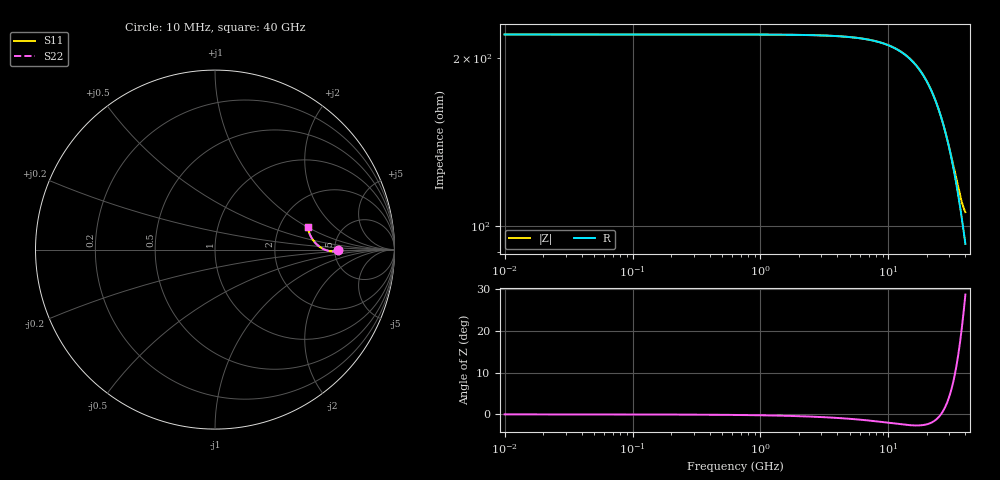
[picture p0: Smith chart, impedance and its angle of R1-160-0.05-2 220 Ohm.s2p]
!version-1
!date-03.2021
# MHz S RI R 50
!Freq ReS11 ImS11 ReS21 ImS21 ReS12 ImS12 ReS22 ImS22
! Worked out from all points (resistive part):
!   801 points, 10 MHz to 40 GHz, reference 50 ohm
!   read as one part in series: R = 220 ohm at 210 MHz
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10  0.6875 -8.09e-06  0.3125 8.07e-06  0.3125 8.07e-06  0.6875 -8.16e-06
3410  0.6864 -0.00274  0.3136 0.00274  0.3136 0.00274  0.6864 -0.00277
6710  0.6834 -0.00532  0.3166 0.0053  0.3166 0.0053  0.6834 -0.00537
10060  0.6779 -0.0077  0.3221 0.00768  0.3221 0.00768  0.6779 -0.00777
13360  0.67 -0.00954  0.33 0.00951  0.33 0.00951  0.67 -0.00963
15060  0.6648 -0.0101  0.3352 0.0101  0.3352 0.0101  0.6648 -0.0103
16710  0.659 -0.0104  0.341 0.0104  0.341 0.0104  0.659 -0.0105
20010  0.6447 -0.0095  0.3553 0.00945  0.3553 0.00945  0.6447 -0.00964
21810  0.6354 -0.00786  0.3646 0.00781  0.3646 0.00781  0.6353 -0.00801
23610  0.6249 -0.00511  0.3751 0.00505  0.3751 0.00505  0.6249 -0.00527
25210  0.6147 -0.00149  0.3853 0.00143  0.3853 0.00143  0.6146 -0.00166
26710  0.6044 0.00313  0.3956 -0.00319  0.3956 -0.00319  0.6043 0.00295
28460  0.5916 0.0103  0.4084 -0.0104  0.4084 -0.0104  0.5915 0.0101
30160  0.5786 0.0195  0.4215 -0.0195  0.4215 -0.0195  0.5785 0.0193
31810  0.5657 0.0307  0.4344 -0.0308  0.4344 -0.0308  0.5655 0.0305
33360  0.5537 0.0437  0.4464 -0.0438  0.4464 -0.0438  0.5535 0.0435
35210  0.5402 0.0624  0.4599 -0.0625  0.4599 -0.0625  0.54 0.0622
36110  0.5342 0.0729  0.4659 -0.073  0.4659 -0.073  0.534 0.0727
37060  0.5284 0.0848  0.4717 -0.085  0.4717 -0.085  0.5282 0.0847
38560  0.5208 0.1056  0.4793 -0.1057  0.4793 -0.1057  0.5206 0.1054
39810  0.5162 0.1245  0.4838 -0.1247  0.4838 -0.1247  0.5161 0.1244
40000  0.5157 0.1275  0.4844 -0.1277  0.4844 -0.1277  0.5155 0.1274
